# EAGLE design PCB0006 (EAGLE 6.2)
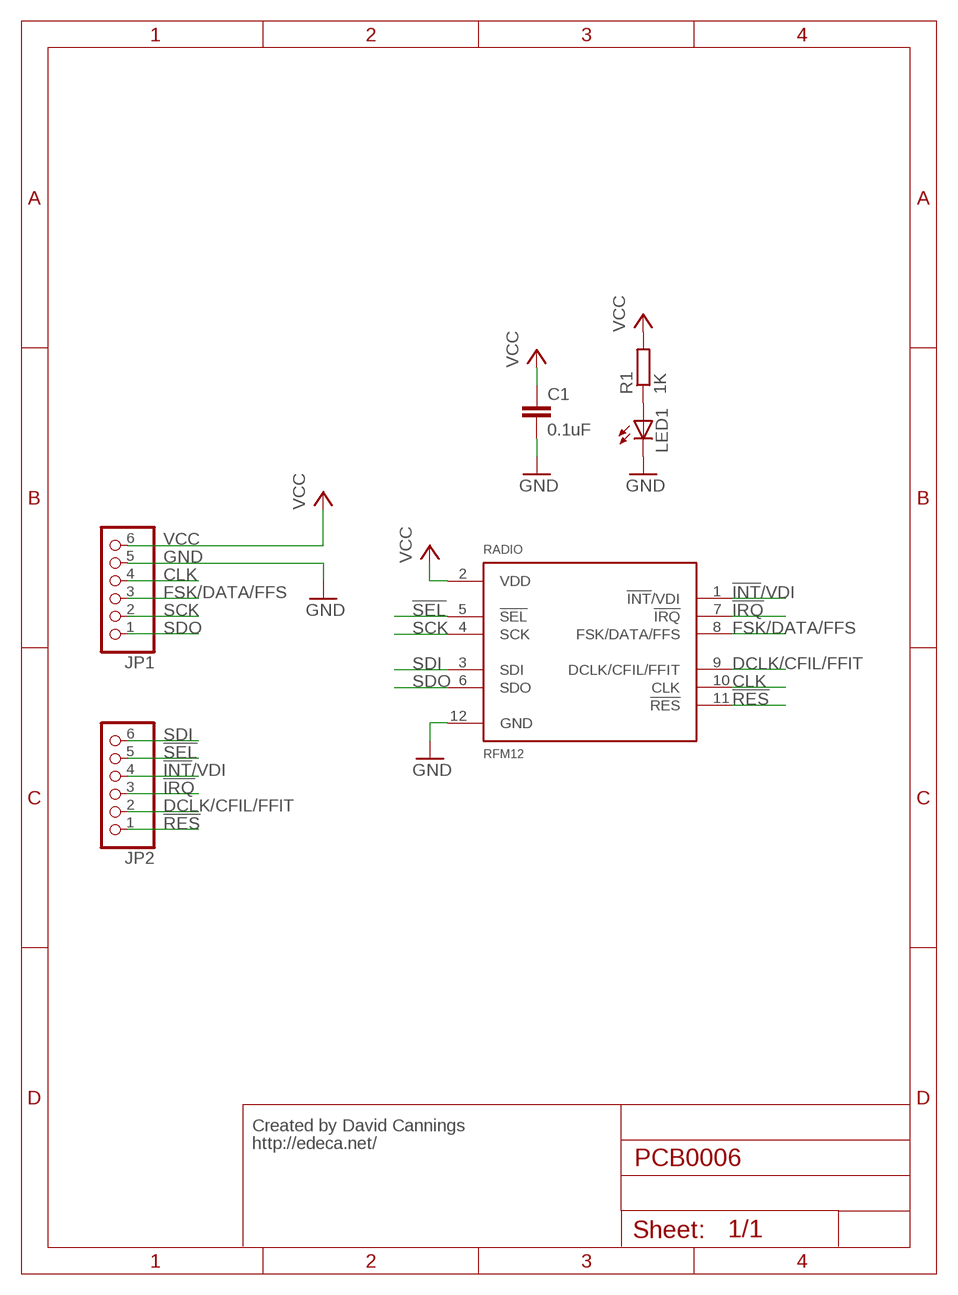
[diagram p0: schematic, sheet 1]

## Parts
C1  0.1uF  C-EU025_050-025X075  [C025_050-025X075]
JP1  PINHD-1X6  [1X06]
JP2  PINHD-1X6  [1X06]
LED1  LED3MM  [LED3MM]
R1  1K  R-EU_0309/V  [0309V]
RADIO  RFM12  [RFM12-PIN]

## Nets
!INT!/VDI: JP2.4 RADIO.1(!INT!/VDI)
!IRQ: JP2.3 RADIO.7(!IRQ)
!RES: JP2.1 RADIO.11(!RES)
!SEL: JP2.5 RADIO.5(!SEL)
CLK: JP1.4 RADIO.10(CLK)
DCLK/CFIL/FFIT: JP2.2 RADIO.9(DCLK/CFIL/FFIT)
FSK/DATA/FFS: JP1.3 RADIO.8(FSK/DATA/FFS)
GND: C1.2 JP1.5 LED1.K(C) RADIO.12(GND)
N$1: LED1.A R1.1
SCK: JP1.2 RADIO.4(SCK)
SDI: JP2.6 RADIO.3(SDI)
SDO: JP1.1 RADIO.6(SDO)
VCC: C1.1 JP1.6 R1.2 RADIO.2(VDD)

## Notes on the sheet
- Created by David Cannings
- http://edeca.net/

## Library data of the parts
C1 = rcl:C-EU: CAPACITOR, European symbol
JP1 JP2 = pinhead:PINHD-1X6: PIN HEADER
LED1 = led:LED: LED
R1 = resistor:R-EU_: RESISTOR, European symbol
RADIO = David's Eagle Library:RFM12; FARNELL_CODE: 1688321; MANUFACTURER: Hirose; MANUFACTURER_CODE: DF11-12DS-2DSA

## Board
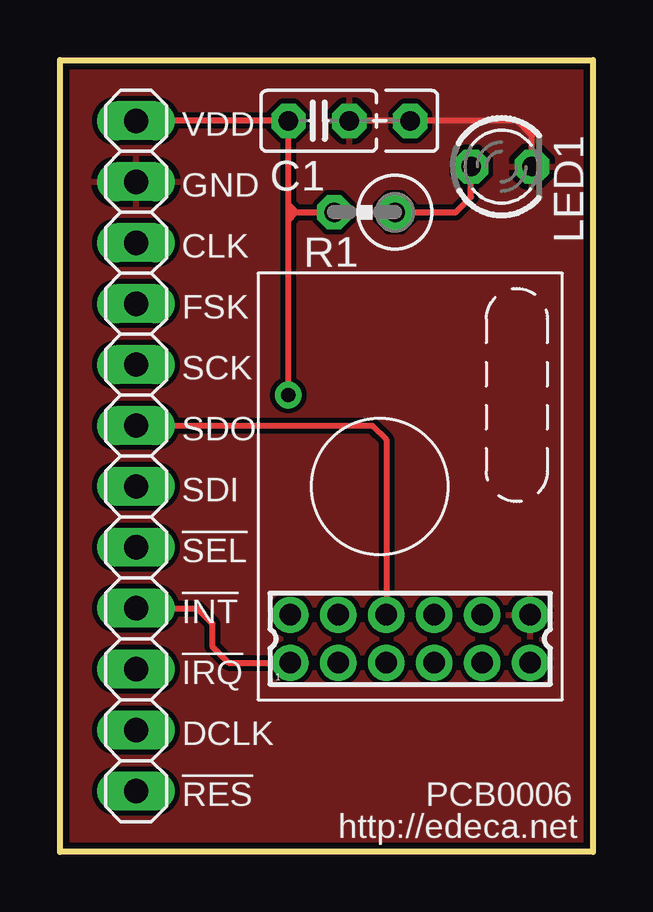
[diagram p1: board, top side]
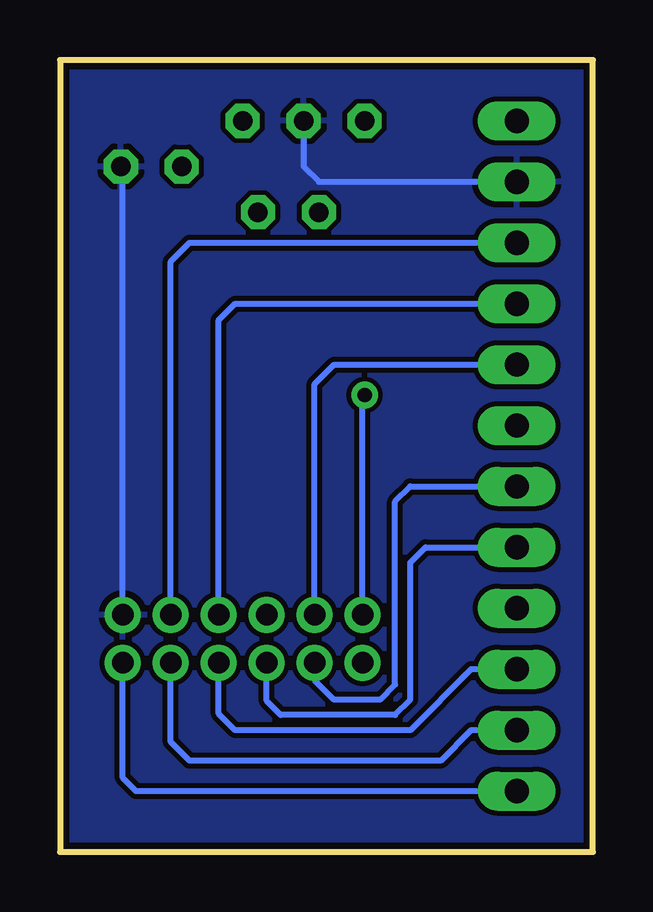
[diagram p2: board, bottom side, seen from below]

Size 22.23 x 33.02 mm. Coordinates in mm from the lower left corner, seen from the top.
Outline: 0,0 0,33.02 22.23,33.02 22.23,0 0,0
Copper layers (1*16): Top 0.035mm / dielectric 1.5mm / Bottom 0.035mm
Design rules: minimum track width 8mil, minimum drill 20mil, track to track 8mil, track to pad 8mil, pad to pad 8mil, via to via 8mil, smd to smd 8mil, copper to edge 10mil, drill to drill 8mil, minimum pad ring 12mil, minimum via ring 10mil, stop-mask expansion 4mil, vias tented up to drill 25mil, thermal gap 10mil

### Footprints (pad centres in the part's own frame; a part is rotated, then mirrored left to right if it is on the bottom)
C025_050-025X075 = drill 0.813 octagon: 1 -1.27,0; 2 1.27,0; 3 3.81,0
1X06 = drill 1.016 long: 1 -6.35,0; 2 -3.81,0; 3 -1.27,0; 4 1.27,0; 5 3.81,0; 6 6.35,0
LED3MM = drill 0.813 octagon: A -1.27,0; K 1.27,0
0309V = drill 0.813 octagon: 1 -1.27,0; 2 1.27,0
RFM12-PIN = drill 0.9 pad 1.27: 1 -5,-1; 2 -5,1; 3 -3,-1; 4 -3,1; 5 -1,-1; 6 -1,1; 7 1,-1; 8 1,1; 9 3,-1; 10 3,1; 11 5,-1; 12 5,1

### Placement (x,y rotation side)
C1  10.79,30.48 0 top
JP1  3.17,24.13 90 top
JP2  3.17,8.89 90 top
LED1  18.41,28.57 0 top
R1  12.7,26.67 180 top
RADIO  14.61,8.89 0 top

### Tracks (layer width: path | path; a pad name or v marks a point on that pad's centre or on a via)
!INT!/VDI
  Top 0.254: JP2.4 5.71,10.16 6.35,9.53 6.35,8.57 7.03,7.89 RADIO.1
!IRQ
  Bottom 0.254: JP2.3 5.08,7.62 7.62,5.08 14.92,5.08 15.61,5.76 RADIO.7
!RES
  Bottom 0.254: RADIO.11 19.61,3.1 19.05,2.54 JP2.1
!SEL
  Bottom 0.254: JP2.5 6.99,12.7 7.62,12.06 7.62,6.35 8.26,5.71 13.02,5.71 13.61,6.3 RADIO.5
CLK
  Bottom 0.254: RADIO.10 17.61,24.62 16.83,25.4 JP1.4
DCLK/CFIL/FFIT
  Bottom 0.254: JP2.2 5.08,5.08 6.35,3.81 16.83,3.81 17.61,4.59 RADIO.9
FSK/DATA/FFS
  Bottom 0.254: RADIO.8 15.61,22.18 14.92,22.86 JP1.3
GND
  Top 0.254: C1.2 19.05,30.48 19.68,29.84 LED1.K
  Bottom 0.254: JP1.5 11.43,27.94 12.06,28.57 C1.2 | RADIO.12 19.61,28.5 LED1.K
  pour Top: 0.64,32.7 21.91,32.7 21.91,0.32 0.32,0.32 0.32,32.7
  pour Bottom: 0.32,32.7 21.91,32.7 21.91,0.32 0.32,0.32
N$1
  Top 0.254: R1.1 16.51,26.67 17.14,27.3 LED1.A
SCK
  Bottom 0.254: JP1.2 10.79,20.32 11.61,19.51 RADIO.4
SDI
  Bottom 0.254: JP2.6 7.62,15.24 8.26,14.61 8.26,6.99 8.89,6.35 10.79,6.35 11.61,7.16 RADIO.3
SDO
  Top 0.254: RADIO.6 13.61,17.19 13.02,17.78 JP1.1
VCC  (via drill 0.6)
  Top 0.254: JP1.6 C1.1 9.53,26.99 | 9.84,26.67 R1.2 | 9.53,26.35 9.84,26.67 | 9.53,26.35 9.53,26.67 | 9.84,26.67 9.53,26.99 | 9.53,26.67 9.53,26.99 | 9.84,26.67 9.53,26.67 | v9.53,19.05 9.53,26.35
  Bottom 0.254: RADIO.2 9.61,18.97 v9.53,19.05

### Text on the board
tPlace: GND | CLK | FSK | SCK | SDO | SDI | !SEL | !INT | !IRQ | DCLK | !RES | http://edeca.net
tNames: VDD | PCB0006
